(* Logix 5000 AddOnInstructionDefinition export ACS_DISABLE_DRIVE; software revision 20.01 *)

ADD_ON_INSTRUCTION ACS_DISABLE_DRIVE   (* revision 2.0, vendor Tolomatic, Inc *)
// Disable ACS Drive
VAR_IN_OUT
   DriveCMD : SINT; {required}   // ToloOutput Reference
END_VAR

ROUTINE Logic   (* ladder *)
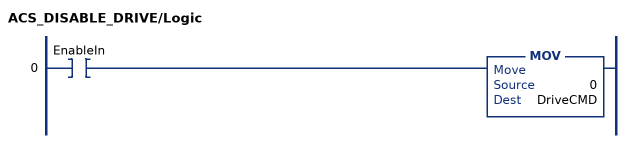
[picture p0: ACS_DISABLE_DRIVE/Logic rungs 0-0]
   0: XIC(EnableIn)MOV(0,DriveCMD);
END_ROUTINE
END_ADD_ON_INSTRUCTION
